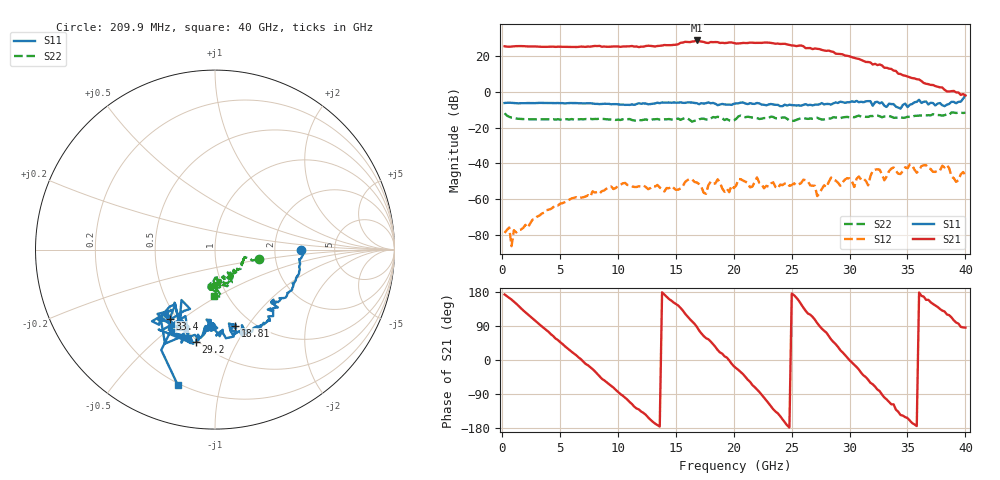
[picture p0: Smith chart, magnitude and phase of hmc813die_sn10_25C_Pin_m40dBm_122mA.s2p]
!Agilent Technologies,E8364C,MY49040264,A.09.00.04
!Agilent E8364C: A.09.00.04
!Date: Tuesday, February 09, 2010 13:51:32
!Correction: S11(Full 2 Port(1,2))
!S21(Full 2 Port(1,2))
!S12(Full 2 Port(1,2))
!S22(Full 2 Port(1,2))
!S2P File: Measurements: S11, S21, S12, S22:
# Hz S  dB  R 50
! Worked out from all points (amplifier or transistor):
!   200 points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, 209.9 MHz to 40 GHz, reference 50 ohm
!   highest |S21| = 28.5 dB at 16.81 GHz (marker M1)
!   |S21| within 3 dB of that: 13.58 GHz to 25.3 GHz (11.72 GHz wide, 60.3 % of centre)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
!   unconditionally stable (mu >= 1): start of sweep to end of sweep
!   at 6.808 GHz: K = 18.77, MAG = 26.3 dB, |S12| = -59.1 dB
!   at 20.2 GHz: K = 7.08, MAG = 28.1 dB, |S12| = -52.3 dB
!   at 40 GHz: K = 49.18, MAG = 2.2 dB, |S12| = -46.4 dB
!   S11 on the Smith chart (normalised r, x): 209.9 MHz: 2.86, -0.02; 18.81 GHz: 0.84, -0.88; 29.2 GHz: 0.48, -0.69; 33.4 GHz: 0.46, -0.45; 40 GHz: 0.19, -0.74
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2.0995e8  -6.34 -0.4  25.29 172.9  -78.72 -129.5  -12.06 -12.8
1.80955e9  -6.46 -7.5  25.36 131.1  -75.98 167.3  -15.30 -14.3
3.40915e9  -6.29 -14.8  24.98 89.0  -68.03 128.6  -15.43 -17.1
5.40865e9  -6.54 -23.5  25.00 36.5  -61.59 88.6  -15.46 -23.6
7.00825e9  -6.56 -30.9  25.02 -4.3  -58.86 53.4  -15.45 -28.8
1.00075e10  -7.05 -42.8  25.20 -84.2  -52.57 0.5  -15.60 -42.3
1.12072e10  -7.14 -43.4  25.43 -116.1  -52.74 -43.2  -15.81 -48.4
1.36066e10  -6.45 -51.4  25.54 -175.7  -53.42 -92.3  -15.59 -53.0
1.540615e10  -5.94 -60.9  27.24 137.3  -53.96 -95.7  -15.75 -54.3
1.68058e10  -6.42 -69.8  28.53 87.9  -50.58 -144.6  -16.24 -56.2
1.740565e10  -6.67 -71.6  27.70 63.0  -56.41 -159.2  -15.07 -62.2
1.88053e10  -7.17 -75.1  27.13 20.1  -50.70 -176.6  -14.23 -73.8
2.020495e10  -6.54 -75.3  26.82 -21.6  -52.33 -145.3  -15.21 -61.0
2.16046e10  -6.78 -86.5  27.30 -66.1  -52.98 -177.7  -14.44 -82.3
2.260435e10  -7.31 -95.6  27.34 -99.0  -53.83 160.4  -14.73 -79.9
2.44039e10  -7.23 -92.5  26.68 -164.9  -51.22 147.5  -14.39 -90.2
2.60035e10  -7.38 -92.9  25.34 138.4  -49.11 140.6  -14.77 -83.0
2.68033e10  -7.69 -92.5  23.70 113.9  -52.43 113.4  -15.10 -82.6
2.92027e10  -5.58 -101.8  20.96 25.9  -52.45 134.8  -14.81 -82.5
3.100225e10  -5.63 -114.9  17.65 -33.8  -49.12 111.7  -13.94 -92.9
3.340165e10  -6.72 -123.2  12.83 -110.5  -44.31 119.7  -13.57 -97.6
4e10  -2.15 -105.5  -2.14 85.5  -46.43 -110.2  -11.76 -91.4
